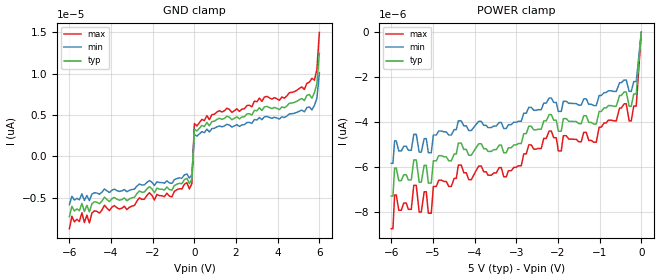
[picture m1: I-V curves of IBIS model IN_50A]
| TEXAS INSTRUMENTS INCORPORATED
| Standard Linear and Logic Group / High Volume Linear
| IBIS Model of TPD4E101
| Four Channel ESD Protection Device
| This file contains package information for the following:
|  QFN 5-pin (DPY) package as [Component] TPD4E101_DPW
| This device can be powered at the following Vccs:
|  5 volt Vcc
| This file provides unique models under the [Model Selector] for each Vcc.
| For operation at a specific Vcc, select the appropriate model after each
| [Model Selector] keyword.
[IBIS Ver]   4.0
[Comment char]  |_char
[File Name]   tpd4e101.ibs
[File Rev]   0 | A1
[Date]   April 17, 2012
[Source]   Data created from TI-SPICE simulations at TI-SLL/HVL.
   The following is an IBIS list for the TPD4E101.
   Please contact sllibis@ti.com with questions and
   comments concerning SLL IBIS models.
[Notes]   Revision_History:
|4
[Disclaimer]
| This model is designed as an aid for customers of Texas Instruments.
| TI and its licensors and suppliers make no warranties, either expressed
| or implied, with respect to this  model, including the warranties of
| merchantability or fitness for a particular purpose. The model is
| provided solely on an "as is" basis. The entire risk as to its quality
| and performance is with the customer.
[Copyright]
| (C) Copyright 2012 Texas Instruments Incorporated. All rights reserved.
| Component TPD4E101_DPW 5-PIN QFN
[Component]   TPD4E101_DPW
[Manufacturer]   Texas Instruments, Inc.
[Package]
|   typ   min   max
R_pkg   3.320e-02   1.030e-03   4.260e-02
L_pkg   2.670e-10   1.450e-11   3.390e-10
C_pkg   9.510e-14   6.530e-14   1.050e-13
[Pin]   signal_name   model_name   R_pin   L_pin   C_pin
1   1   IN_50A   4.260e-02   3.190e-10   1.020e-13
2   2   IN_50A   4.080e-02   3.390e-10   1.050e-13
3   3   IN_50A   4.060e-02   3.320e-10   1.020e-13
4   4   IN_50A   4.080e-02   3.330e-10   1.010e-13
5   5   GND   1.030e-03   1.450e-11   7.530e-14
| Models and submodels in the file (1): IN_50A (Input)
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| Model IN
[Model]   IN_50A
Model_type  Input
Vinl=0
Vinh=5
| variable   typ   min   max
|   slow   nom   fast
C_comp   4.7pF   3.9pF   5.8pF
[Temperature Range]   40   100   -40
| Ambient temperature   25   85   -40
[Voltage range]   5   5   5
[GND Clamp]
| IN_50A
|   Voltage   I(typ)   I(min)   I(max)
-6V       -7.29pA    -5.83pA    -8.74pA
-5.88V    -6.04pA    -4.83pA    -7.24pA
-5.04V    -6.71pA    -5.36pA    -8.05pA
-4.32V    -4.93pA    -3.94pA    -5.91pA
-3.24V    -5.36pA    -4.28pA    -6.43pA
-240mV    -3.29pA    -2.63pA    -3.94pA
-120mV    -2.74pA    -2.19pA    -3.28pA
0V        3.32pA     2.65pA     3.98pA
5.28V     6.75pA     5.4pA      8.1pA
5.76V     7.69pA     6.15pA     9.22pA
5.88V     8.8pA      7.04pA     10.5pA
6V        12.5pA     10.1pA     15pA
[POWER Clamp]
| IN_50A
|   Voltage   I(typ)   I(min)   I(max)
-6V       -7.29pA    -5.83pA    -8.74pA
-5.92V    -6.04pA    -4.83pA    -7.24pA
-5.4V     -5.68pA    -4.54pA    -6.81pA
-5.04V    -6.71pA    -5.36pA    -8.05pA
-4.99V    -5.72pA    -4.57pA    -6.86pA
-4.39V    -4.93pA    -3.94pA    -5.91pA
-3.24V    -5.36pA    -4.28pA    -6.43pA
-2.21V    -3.66pA    -2.92pA    -4.39pA
-1.92V    -4.4pA     -3.52pA    -5.28pA
-240mV    -3.29pA    -2.63pA    -3.94pA
-120mV    -2.74pA    -2.19pA    -3.28pA
0V        0A         0A         0A
